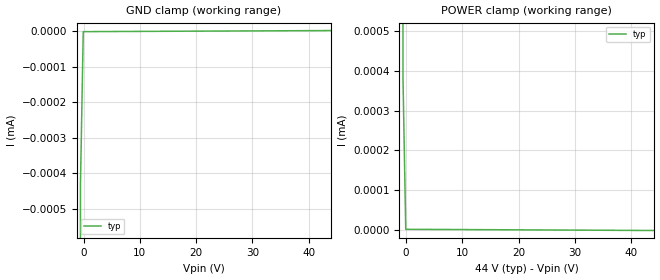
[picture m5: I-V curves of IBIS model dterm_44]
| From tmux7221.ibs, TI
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| dterm_44
[Model]   dterm_44
Model_type   Terminator
|   typ   min   max
C_comp   1.598234e-11   NA   NA
[Voltage Range]   44   NA   NA
[Temperature Range]   27   NA   NA
[Power Clamp Reference]   44   NA   NA
[GND Clamp Reference]   0   NA   NA
[GND Clamp]
|   Voltage   I(typ)   I(min)   I(max)
-5V       -4.891A    NA         NA
-1.04V    -82.6mA    NA         NA
-545.5mV  -431.2nA   NA         NA
-50.51mV  -1.525nA   NA         NA
44V       1.52nA     NA         NA
[POWER Clamp]
|   Voltage   I(typ)   I(min)   I(max)
-5V       5.384A     NA         NA
-1.04V    81.53mA    NA         NA
-545.5mV  385.6nA    NA         NA
-50.5mV   1.524nA    NA         NA
44V       -1.521nA   NA         NA
